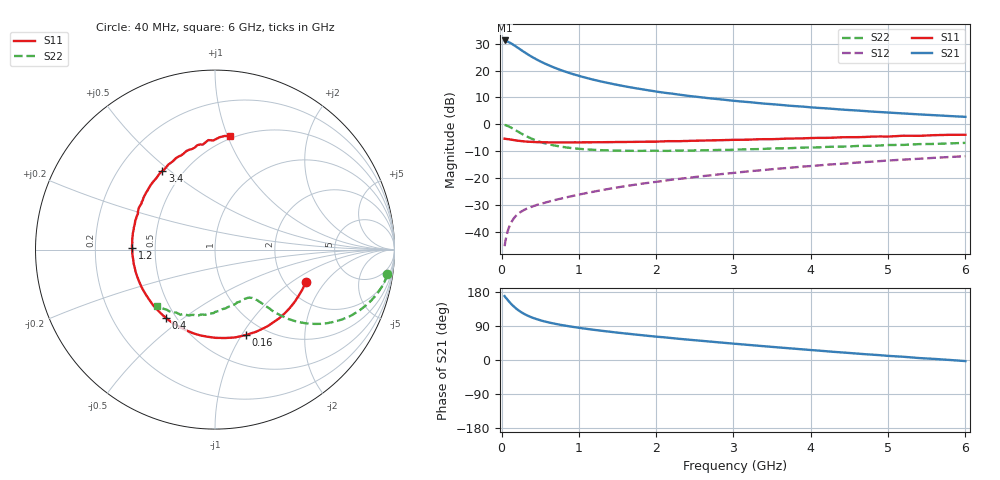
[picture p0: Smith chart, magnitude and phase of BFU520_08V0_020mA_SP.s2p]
! Filename:  P:\Prog\Test\Noise\ATS_data\Testdata_Net\03 Spar\BFU520_APG2013_37_A05_08p0V_020mA_SP_CM01_D.s2p
! Date/Time: Fri 26/Apr/2013 13:00:10
! BFU520_APG2013_37_A05_08p0V_1to20mA_SP_CM01_Bias8_R.s2p
! MDIF S-parameter v. bias file
! BFU520_APG2013_37_A05_08p0V_1to20mA_SP_CM01
! Date/time Tue Apr 23 17:06:44 2013
! VAR V_out= 8.0000
! VAR I_out= 19.9900
! VAR V_in= 0.8221
! VAR I_in= 0.2227
! Device data file deembeded for feedlines and parallel
! Original file: \03 Spar\BFU520_APG2013_37_A05_08p0V_020mA_SP_CM01_R.s2p
! Feed-files: PR047V01_250413_Feed1.s2p, PR047V01_250413_Feed2.s2p
! Parallel-file: PR047V01_250413_Par.s2p
# MHz S MA R 50
!  Freq-MHz  S11-mag  S11-arg  S21-mag  S21-arg  S12-mag  S12-arg  S22-mag  S22-arg
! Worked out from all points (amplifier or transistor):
!   98 points, 40 MHz to 6 GHz, reference 50 ohm
!   highest |S21| = 31.2 dB at 40 MHz (marker M1)
!   |S21| within 3 dB of that: start of sweep to 225.2 MHz
!   unconditionally stable (mu >= 1): 1.379 GHz to 3.434 GHz
!   at 300 MHz: K = 0.46, MSG = 29.3 dB, |S12| = -31.8 dB
!   at 1.6 GHz: K = 1.03, MAG = 17.6 dB, |S12| = -23.1 dB
!   at 6 GHz: K = 0.83, MSG = 7.3 dB, |S12| = -11.9 dB
!   S11 on the Smith chart (normalised r, x): 40 MHz: 2.59, -1.31; 160 MHz: 0.81, -1.04; 400 MHz: 0.44, -0.43; 1.2 GHz: 0.37, +0.01; 3.4 GHz: 0.39, +0.47; 6 GHz: 0.48, +1.02
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40  0.5386 -19.5  36.4 168.6  0.00535 82.3  0.9693 -8.2
50  0.5352 -24.4  36.29 165.4  0.00663 80.4  0.9632 -10.3
90  0.5262 -42.6  34.05 155.9  0.01124 74.1  0.9158 -18.0
120  0.518 -55.4  32.38 149.0  0.01429 69.8  0.8714 -23.1
160  0.506 -70.4  29.74 141.0  0.0177 65.0  0.8093 -28.7
180  0.502 -77.2  28.49 137.5  0.0192 63.2  0.778 -31.1
220  0.4919 -89.3  26.09 131.0  0.02169 60.1  0.7195 -35.1
280  0.4821 -104.2  22.76 123.1  0.02477 57.1  0.6427 -39.5
340  0.4726 -116.2  20.04 116.8  0.02719 55.4  0.5812 -42.5
400  0.4683 -125.9  17.79 111.7  0.02935 54.7  0.5314 -44.5
500  0.4632 -138.5  14.88 105.0  0.0327 54.4  0.4708 -46.7
650  0.4594 -152.3  11.88 97.3  0.03744 55.3  0.412 -48.5
850  0.4593 -165.0  9.297 89.8  0.04383 57.0  0.3679 -50.1
1050  0.4599 -175.0  7.621 83.5  0.05052 58.5  0.3445 -52.1
1200  0.4619 179.0  6.706 79.5  0.0557 59.4  0.3335 -53.7
1600  0.4673 165.5  5.071 70.0  0.07004 60.4  0.3209 -58.9
2050  0.4774 154.2  3.968 60.8  0.08627 60.3  0.3199 -66.1
3100  0.5137 130.2  2.655 41.5  0.1282 57.0  0.3391 -84.5
3400  0.5275 123.8  2.42 36.3  0.1406 55.3  0.3477 -90.0
4100  0.557 111.3  2.016 24.8  0.1708 51.0  0.3709 -102.4
5200  0.6114 93.5  1.588 8.5  0.2193 42.7  0.4122 -121.8
6000  0.6365 82.4  1.374 -2.8  0.254 35.8  0.4497 -135.5
